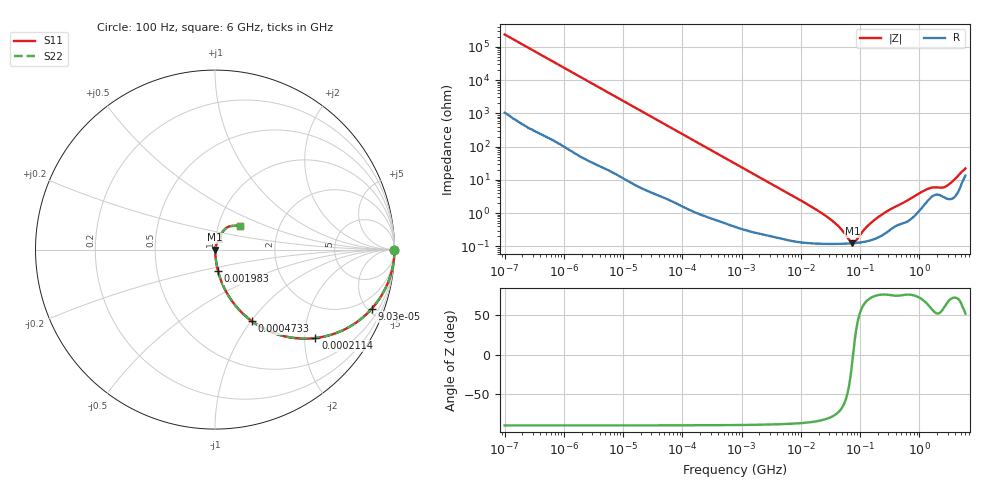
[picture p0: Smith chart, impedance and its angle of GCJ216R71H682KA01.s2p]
!Murata Part Number: GCJ216R71H682KA01
!These Parameters are Measured in Series Mode Connection
!Data Generated on Mar 13, 2026
!  o--ll--o
!Port1  Port2
!  o------o
!Operation Temp=25[degC], DC Bias Voltage=0[V]
!Freq. Start=100[Hz] Stop=6[GHz] 401[Steps]
# Hz S RI R 50
!Freq.(Hz) S11(Real) S11(Imag) S21(Real) S21(Imag) S12(Real) S12(Imag) S22(Real) S22(Imag)
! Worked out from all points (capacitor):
!   401 points, 100 Hz to 6 GHz, reference 50 ohm
!   read as one part in series: C = 6.81 nF near 109 Hz
!   lowest |Z| = 125 mohm at 74.56 MHz (marker M1)
!   series resonance near 76.2 MHz, so ESL is about 640 pH
!   S11 on the Smith chart (normalised r, x): 100 Hz: open; 90.3 kHz: 1.03, -5.27; 211.4 kHz: 1.02, -2.26; 473.3 kHz: 1.01, -1.01; 1.983 MHz: 1.00, -0.24; 6 GHz: 1.27, +0.35
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100  1 -0.000429  2.1e-06 0.000429  2.1e-06 0.000429  1 -0.000429
2008  0.9999 -0.00854  0.000107 0.00854  0.000107 0.00854  0.9999 -0.00854
12592  0.9969 -0.0531  0.00308 0.0531  0.00308 0.0531  0.9969 -0.0531
40335  0.971 -0.165  0.029 0.165  0.029 0.165  0.971 -0.165
90302  0.8724 -0.3304  0.1276 0.3304  0.1276 0.3304  0.8724 -0.3304
211427  0.5597 -0.4926  0.4403 0.4926  0.4403 0.4926  0.5597 -0.4926
473344  0.2063 -0.3994  0.7937 0.3994  0.7937 0.3994  0.2063 -0.3994
774597  0.0906 -0.2808  0.9094 0.2808  0.9094 0.2808  0.0906 -0.2808
1983483  0.0169 -0.1193  0.9831 0.1193  0.9831 0.1193  0.0169 -0.1193
1.555665e7  0.00146 -0.0151  0.9985 0.0151  0.9985 0.0151  0.00146 -0.0151
3.80911e7  0.00121 -0.00482  0.9988 0.00482  0.9988 0.00482  0.00121 -0.00482
4.983056e7  0.00121 -0.00281  0.9988 0.00281  0.9988 0.00281  0.00121 -0.00281
6.817316e7  0.00123 -0.000715  0.9988 0.000715  0.9988 0.000715  0.00123 -0.000715
7.455971e7  0.00124 -0.000138  0.9988 0.000138  0.9988 0.000138  0.00124 -0.000138
8.527865e7  0.00127 0.000727  0.9987 -0.000727  0.9987 -0.000727  0.00127 0.000727
1.166697e8  0.00137 0.00282  0.9986 -0.00282  0.9986 -0.00282  0.00137 0.00282
1.526266e8  0.00155 0.00484  0.9984 -0.00484  0.9984 -0.00484  0.00155 0.00484
3.124326e8  0.00316 0.0121  0.9968 -0.0121  0.9968 -0.0121  0.00316 0.0121
1.369159e9  0.0244 0.0455  0.9756 -0.0455  0.9756 -0.0455  0.0244 0.0455
2.802721e9  0.0302 0.0535  0.9698 -0.0535  0.9698 -0.0535  0.0302 0.0535
4.193612e9  0.0444 0.1012  0.9556 -0.1012  0.9556 -0.1012  0.0444 0.1012
6e9  0.1388 0.1322  0.8612 -0.1322  0.8612 -0.1322  0.1388 0.1322
